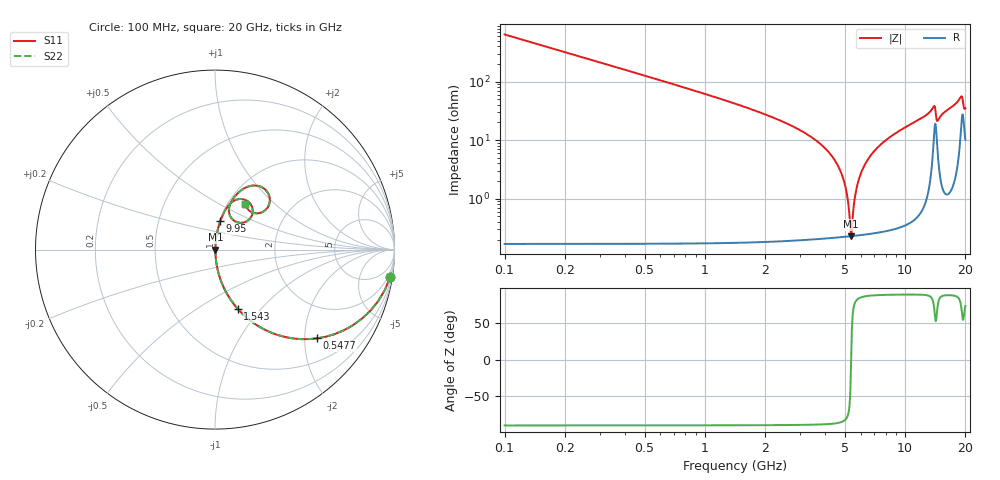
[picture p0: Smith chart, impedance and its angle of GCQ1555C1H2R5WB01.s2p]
!Murata Part Number: GCQ1555C1H2R5WB01
!These Parameters are Measured in Series Mode Connection
!Data Generated on Mar 13, 2026
!  o--ll--o
!Port1  Port2
!  o------o
!Operation Temp=25[degC], DC Bias Voltage=0[V]
!Freq. Start=100[MHz] Stop=20[GHz] 401[Steps]
# Hz S RI R 50
!Freq.(Hz) S11(Real) S11(Imag) S21(Real) S21(Imag) S12(Real) S12(Imag) S22(Real) S22(Imag)
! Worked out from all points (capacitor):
!   401 points, 100 MHz to 20 GHz, reference 50 ohm
!   read as one part in series: C = 2.5 pF near 199.5 MHz
!   lowest |Z| = 229 mohm at 5.373 GHz (marker M1)
!   series resonance near 5.377 GHz, so ESL is about 350 pH
!   S11 on the Smith chart (normalised r, x): 100 MHz: 1, -13; 547.8 MHz: 1.00, -2.30; 1.543 GHz: 1.00, -0.76; 9.95 GHz: 1.01, +0.33; 20 GHz: 1.20, +0.67
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1e8  0.9759 -0.1533  0.0241 0.1533  0.0241 0.1533  0.9759 -0.1533
2.99e8  0.8182 -0.3853  0.1818 0.3853  0.1818 0.3853  0.8182 -0.3853
5.4775e8  0.5694 -0.4944  0.4306 0.4944  0.4306 0.4944  0.5694 -0.4944
9.955e8  0.2767 -0.446  0.7233 0.446  0.7233 0.446  0.2767 -0.446
1.54275e9  0.1267 -0.3303  0.8733 0.3303  0.8733 0.3303  0.1267 -0.3303
3.43325e9  0.0139 -0.1085  0.9861 0.1085  0.9861 0.1085  0.0139 -0.1085
4.7765e9  0.00299 -0.0282  0.997 0.0282  0.997 0.0282  0.00299 -0.0282
5.075e9  0.00242 -0.0138  0.9976 0.0138  0.9976 0.0138  0.00242 -0.0138
5.3735e9  0.00228 -0.000173  0.9977 0.000173  0.9977 0.000173  0.00228 -0.000173
5.473e9  0.00231 0.0042  0.9977 -0.0042  0.9977 -0.0042  0.00231 0.0042
5.672e9  0.00249 0.0127  0.9975 -0.0127  0.9975 -0.0127  0.00249 0.0127
5.871e9  0.0028 0.021  0.9972 -0.021  0.9972 -0.021  0.0028 0.021
6.7665e9  0.00559 0.0554  0.9944 -0.0554  0.9944 -0.0554  0.00559 0.0554
9.9505e9  0.029 0.1576  0.971 -0.1576  0.971 -0.1576  0.029 0.1576
1.005e10  0.0301 0.1605  0.9699 -0.1605  0.9699 -0.1605  0.0301 0.1605
1.338325e10  0.1035 0.2711  0.8965 -0.2711  0.8965 -0.2711  0.1035 0.2711
1.398025e10  0.1986 0.2533  0.8014 -0.2533  0.8014 -0.2533  0.1986 0.2533
1.447775e10  0.1008 0.1654  0.8992 -0.1654  0.8992 -0.1654  0.1008 0.1654
1.67165e10  0.1176 0.3044  0.8824 -0.3044  0.8824 -0.3044  0.1176 0.3044
1.895525e10  0.2742 0.3391  0.7258 -0.3391  0.7258 -0.3391  0.2742 0.3391
1.95025e10  0.2514 0.2042  0.7486 -0.2042  0.7486 -0.2042  0.2514 0.2042
2e10  0.1696 0.2539  0.8304 -0.2539  0.8304 -0.2539  0.1696 0.2539
